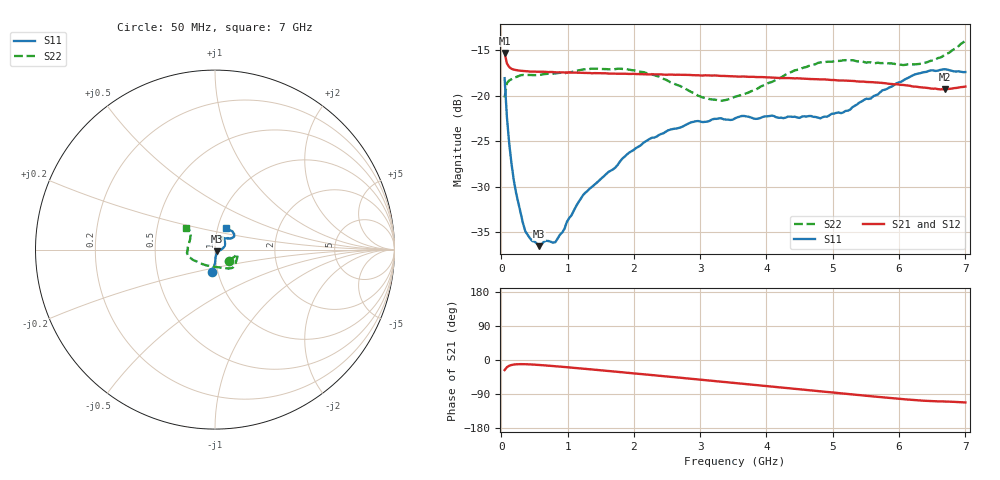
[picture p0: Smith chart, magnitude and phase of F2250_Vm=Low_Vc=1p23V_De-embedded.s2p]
! Integrated Device Technology
! Corporate Headquarters
! 6024 Silver Creek Valley Road
! San Jose, CA 95138  USA
! Phone:  1-408-284-8200
! Toll Free:  1-800-223-1366
! Webpage:  http://www.idt.com/
! Timing and RF Division
! 515 Groton Road, Suite 102
! Westford, MA 01886-6024
! Device:  F2250
! Description: Voltage Variable RF Attenuator
! Frequency:  50.0 -  6000.00 MHz
! Package:  3x3 mm Thin QFN Plastic Package: 16 pin
! Ports:  2 RF, 3 DC
!  Pin  1  = GND
!  Pin  2  = NC
!  Pin  3  = RF1  = Port 1
!  Pin  4  = NC
!  Pin  5  = GND
!  Pin  6  = GND
!  Pin  7  = GND
!  Pin  8  = GND
!  Pin  9  = NC
!  Pin 10  = RF2  = Port 2
!  Pin 11  = NC
!  Pin 12  = GND
!  Pin 13  = GND
!  Pin 14  = VCNTRL
!  Pin 15  = VDD
!  Pin 16  = VMODE
! Vcntrl:  1.230 Volts
! Vmode:  +0.000 Volts
! Vdd:  +3.30  Volts
! Current:  1.191 mA
! Data:  The device was measured on a the F2250 evaluation board which has
!  individual transmission lines to the RF pins.  Data was collected
!  using a calibrated network analyzer.  The evaluation board was
!  de-embedded using a TRL calibration technique.
!  The reference plane is the edge of the package pin.
! Misc:  SN 10
!  Action Tracker AT0258
! Date Measured:  2014-11-26
! Date:  2015-10-15  MJV
! Note:
!  Integrated Device Technology supplies this data as a sample of measured
!  data at the package pin for this product.  Your particular data for this
!  product may vary.
!  Data was taken at 25 degrees C.
!  Integrated Device Technology reserves the right to change this data at anytime.
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# GHz S dB R 50
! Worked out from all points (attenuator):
!   201 points, 50 MHz to 7 GHz, reference 50 ohm
!   highest |S21| = -15.27 dB at 50 MHz (marker M1); lowest = -19.3 dB at 6.687 GHz (marker M2)
!   lowest |S11| = -36.5 dB at 571.2 MHz (marker M3), VSWR 1.03, Z = 51.2 - j0.868 ohm
!   |S11| at or under -10 dB: start of sweep to end of sweep
!   |S22| runs from -20.5 to -13.9 dB; largest |S21 - S12| = 0.0006
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0.05  -18.04 -97.7  -15.27 -26.5  -15.26 -26.5  -20.16 -38.9
0.08475  -22.32 -89.8  -16.42 -19.0  -16.42 -19.0  -18.59 -18.8
0.1195  -25.23 -87.5  -16.82 -15.2  -16.83 -15.2  -18.30 -13.7
0.189  -29.28 -81.1  -17.11 -12.0  -17.10 -12.0  -17.99 -11.8
0.22375  -30.68 -75.9  -17.15 -11.4  -17.16 -11.4  -17.92 -12.2
0.36275  -34.88 -60.6  -17.26 -11.1  -17.27 -11.1  -17.71 -13.1
0.57125  -36.51 -34.5  -17.34 -13.1  -17.33 -13.1  -17.68 -18.3
0.6755  -35.92 -30.8  -17.36 -14.5  -17.36 -14.5  -17.58 -21.0
0.8145  -36.07 -19.8  -17.40 -16.4  -17.40 -16.4  -17.53 -25.0
1.2315  -30.92 -7.4  -17.46 -22.8  -17.46 -22.8  -17.09 -34.8
1.9265  -26.23 13.4  -17.58 -33.9  -17.56 -34.0  -17.10 -46.7
2.37825  -24.29 24.8  -17.63 -41.4  -17.61 -41.4  -17.87 -55.7
2.86475  -22.89 40.2  -17.71 -49.6  -17.71 -49.6  -19.56 -73.0
3.0385  -22.87 46.6  -17.75 -52.5  -17.72 -52.5  -20.16 -82.3
3.3165  -22.44 55.6  -17.80 -57.2  -17.78 -57.3  -20.52 -101.0
3.525  -22.46 60.5  -17.85 -60.8  -17.83 -60.8  -20.09 -115.2
4.7065  -22.29 66.7  -18.15 -80.9  -18.13 -80.9  -16.57 -162.8
5.22775  -21.62 49.5  -18.32 -89.8  -18.32 -89.8  -16.08 -172.7
5.85325  -19.06 34.7  -18.67 -100.1  -18.65 -100.2  -16.43 173.4
6.305  -17.52 36.7  -19.03 -106.6  -19.02 -106.7  -16.48 157.8
6.68725  -17.06 46.3  -19.28 -109.5  -19.26 -109.6  -15.46 144.5
7  -17.37 63.1  -18.96 -112.1  -18.96 -112.2  -13.90 142.4
